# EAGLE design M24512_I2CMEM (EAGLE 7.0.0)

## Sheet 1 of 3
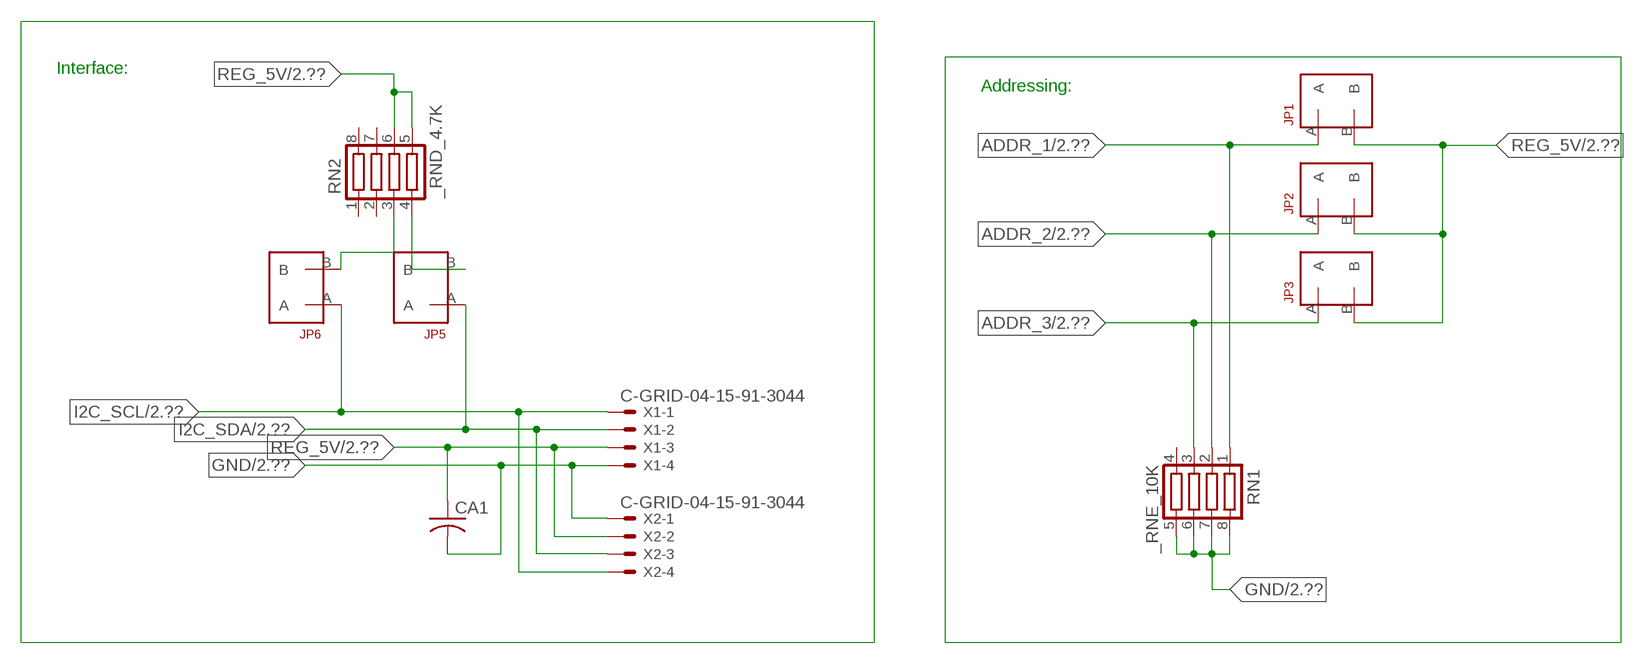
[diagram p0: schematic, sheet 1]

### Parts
CA1  CC1206KRX7R9BB104  [.1UF]
JP1  JUMPER_1X2_2MM  [JUMPER_1X2_2MM]
JP2  JUMPER_1X2_2MM  [JUMPER_1X2_2MM]
JP3  JUMPER_1X2_2MM  [JUMPER_1X2_2MM]
JP5  JUMPER_1X2_2MM  [JUMPER_1X2_2MM]
JP6  JUMPER_1X2_2MM  [JUMPER_1X2_2MM]
RN1  _RNE_10K  [RNE]
RN2  _RND_4.7K  [RND]
X1  C-GRID-04-15-91-3044  [15-91-04]
X2  C-GRID-04-15-91-3044  [15-91-04]

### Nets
ADDR_1: JP1.A RN1.1 ; also sheet 2
ADDR_2: JP2.A RN1.2 ; also sheet 2
ADDR_3: JP3.A RN1.3 ; also sheet 2
GND: CA1.2 RN1.5 RN1.6 RN1.7 RN1.8 X1.4 X2.1 ; also sheet 2,3
I2C_SCL: JP6.A X1.1 X2.4 ; also sheet 2
I2C_SDA: JP5.A X1.2 X2.3 ; also sheet 2
N$1: JP6.B RN2.3
N$2: JP5.B RN2.4
REG_5V: CA1.1 JP1.B JP2.B JP3.B RN2.5 RN2.6 X1.3 X2.2 ; also sheet 2,3
Unconnected: RN1.4 RN2.1 RN2.2 RN2.7 RN2.8

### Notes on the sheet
- Interface:
- Addressing:

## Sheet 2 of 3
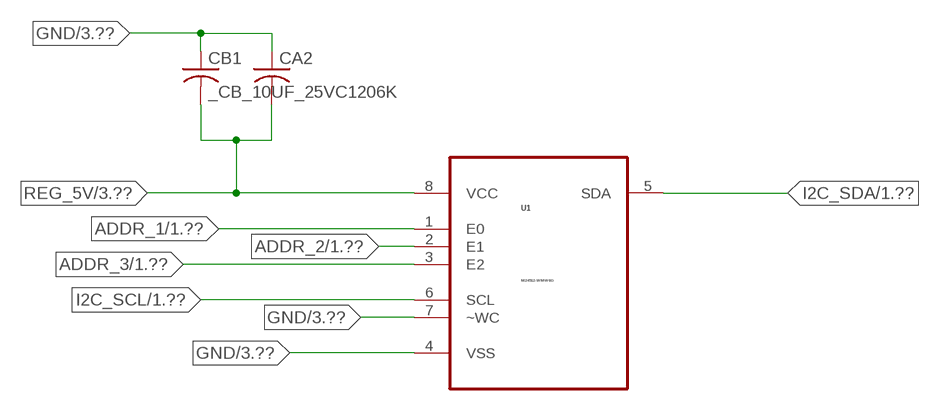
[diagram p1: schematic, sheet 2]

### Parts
CA2  _CA_.10UF_50VC1206K  [_CA_.1UF_50V]
CB1  _CB_10UF_25VC1206K  [_CB_10UF_25V]
U1  M24512-WMW6G  [SOIC127P825X250-8N]

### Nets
ADDR_1: U1.1(E0) ; also sheet 1
ADDR_2: U1.2(E1) ; also sheet 1
ADDR_3: U1.3(E2) ; also sheet 1
GND: CA2.1 CB1.1 U1.4(VSS) U1.7(~WC) ; also sheet 1,3
I2C_SCL: U1.6(SCL) ; also sheet 1
I2C_SDA: U1.5(SDA) ; also sheet 1
REG_5V: CA2.2 CB1.2 U1.8(VCC) ; also sheet 1,3

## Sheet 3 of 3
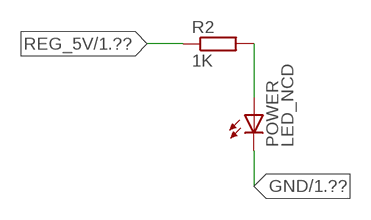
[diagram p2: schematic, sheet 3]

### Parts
POWER  LED_NCD  [CHIPLED_0603]
R2  1K  RESISTOR_SMT-0402  [R402]

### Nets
GND: POWER.C ; also sheet 1,2
N$13: POWER.A R2.2
REG_5V: R2.1 ; also sheet 1,2

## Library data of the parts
CA1 = NCD_ULTIMATE_LIBRARY:CC1206KRX7R9BB104: Capacitor CA .1uF 50V SMT C1206K CC1206KRX7R9BB104
CA2 = NCD_ULTIMATE_LIBRARY:_CA_.10UF_50V: Capacitor .1uF SMT
CB1 = NCD_ULTIMATE_LIBRARY:_CB_10UF_25V: Capacitor 10uF SMT
JP1-JP3 JP5 JP6 = NCD_ULTIMATE_CONNECTORS:JUMPER_1X2_2MM
POWER = NCD_ULTIMATE_LIBRARY:LED_NCD: LED Digikey 754-1132-2-ND/APT2012SRCPRV
R2 = NCD_ULTIMATE_LIBRARY:RESISTOR_SMT: NCD Resistor
RN1 = NCD_ULTIMATE_LIBRARY:_RNE_10K: Resistor Array RNE SMT 10K x 4 Single Resistor Source: http://www.ctscorp.com/components/Datasheets/CTSChipArrayDs.pdf Digikey 742C083103JPTR-ND/742C083103JP; OC_FARNELL: unknown; OC_NEWARK: unknown
RN2 = NCD_ULTIMATE_LIBRARY:_RND_4.7K: Resistor Array RND SMT 4.7K x 4 Single Resistor Source: http://www.ctscorp.com/components/Datasheets/CTSChipArrayDs.pdf Digikey 742C083472JPTR-ND/742C083472JP; OC_FARNELL: unknown; OC_NEWARK: unknown
U1 = NCD_ULTIMATE_bhaskar:M24512-WMW6G: Digikey 497-8625-6-ND/M24512-WDW6TP; MPN: M24512-WMW6G; OC_FARNELL: 1099661; OC_NEWARK: 56P9161; PACKAGE: SOIC-8; SUPPLIER: STMICROELECTRONICS
X1 X2 = NCD_ULTIMATE_CONNECTORS:C-GRID-04: CONNECTOR 4-Pos I2C wire to board 2.54 mm (0.100") pitch header Digikey WM1342-ND/0015912045; OC_FARNELL: unknown; OC_NEWARK: unknown

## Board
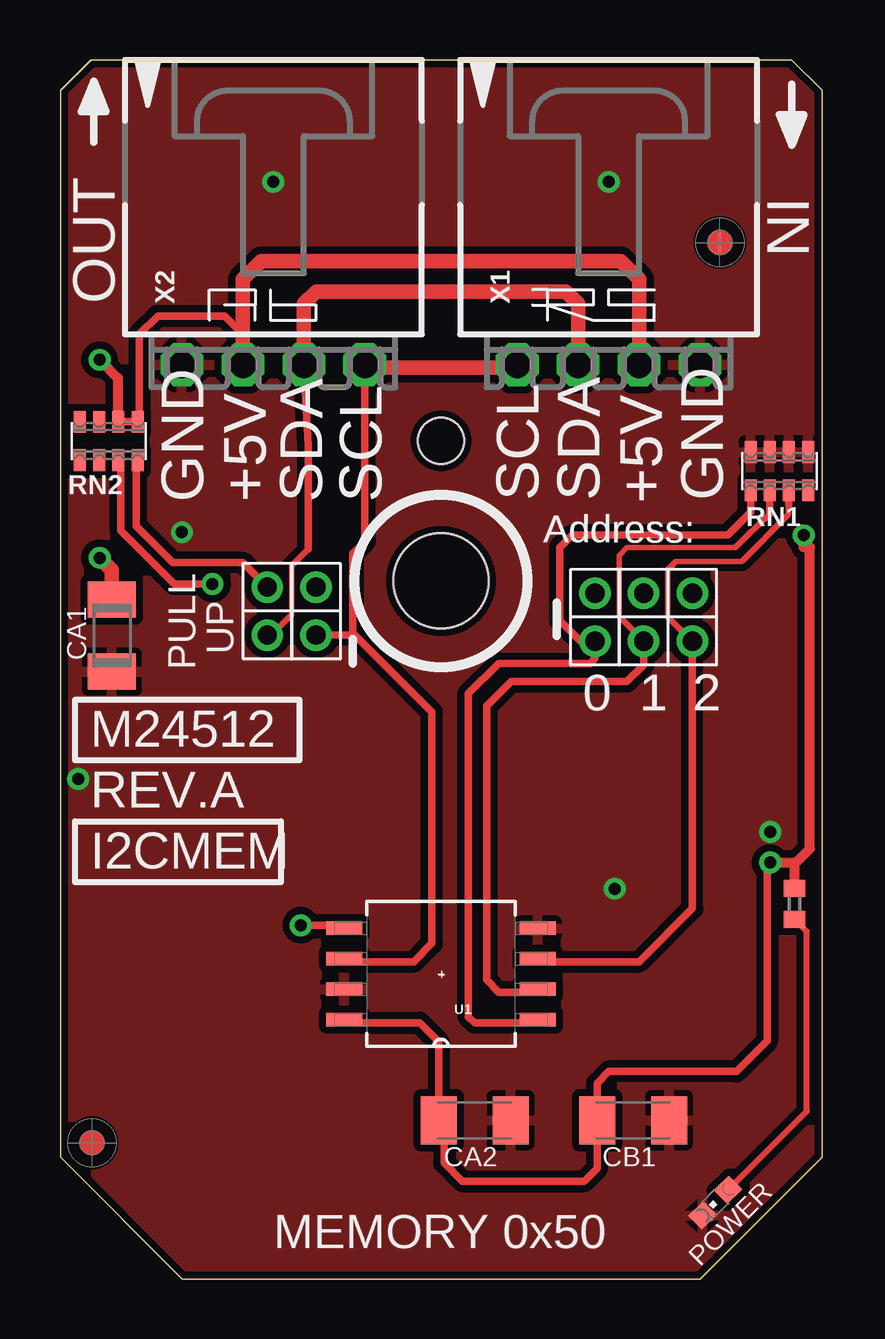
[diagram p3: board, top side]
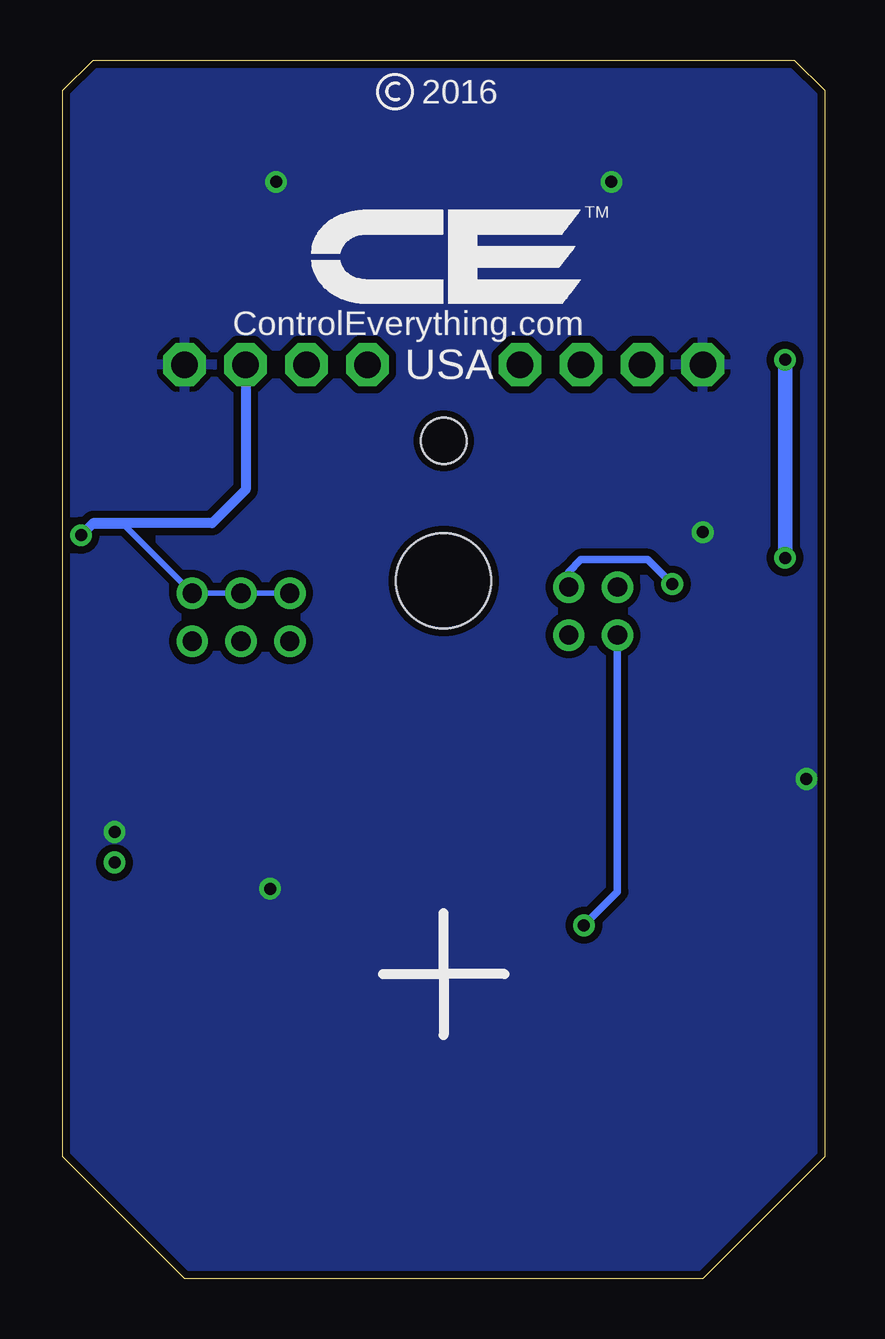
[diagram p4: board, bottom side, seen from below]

Size 31.75 x 50.8 mm. Coordinates in mm from the lower left corner, seen from the top.
Outline: 32 segments
Copper layers (1*16): Top 0.035mm / dielectric 1.5mm / Bottom 0.035mm
Design rules "default": minimum track width 5mil, minimum drill 24mil, track to track 5mil, track to pad 5mil, pad to pad 5mil, via to via 5mil, smd to smd 5mil, copper to edge 10mil, drill to drill 8mil, minimum pad ring 10mil, minimum via ring 8mil, stop-mask expansion 2mil, vias tented up to drill 0mil, thermal gap 10mil
Holes 3.96 mm at 15.88,29.08
Holes 1.91 mm at 15.88,34.92

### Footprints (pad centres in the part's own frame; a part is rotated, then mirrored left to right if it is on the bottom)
.1UF = smd 1.5 x 2: 1 -1.5,0; 2 1.5,0
_CA_.1UF_50V = smd 1.5 x 2: 1 -1.5,0; 2 1.5,0
_CB_10UF_25V = smd 1.5 x 2: 1 -1.5,0; 2 1.5,0
JUMPER_1X2_2MM = drill 0.8: A 0,2; B 0,0
CHIPLED_0603 = smd 0.8 x 0.876: A 0,-0.75; C 0,0.75
R402 = smd 0.7 x 0.9: 1 -0.65,0; 2 0.65,0
RNE = smd 0.5 x 0.9: 1 -1.2,-0.8; 2 -0.4,-0.8; 3 0.4,-0.8; 4 1.2,-0.8; 5 1.2,0.8; 6 0.4,0.8; 7 -0.4,0.8; 8 -1.2,0.8
RND = smd 0.5 x 0.9: 1 -1.2,-0.8; 2 -0.4,-0.8; 3 0.4,-0.8; 4 1.2,-0.8; 5 1.2,0.8; 6 0.4,0.8; 7 -0.4,0.8; 8 -1.2,0.8
SOIC127P825X250-8N = smd 1.499 x 0.559: 1 -4.039,1.905; 2 -4.039,0.635; 3 -4.039,-0.635; 4 -4.039,-1.905; 5 4.039,-1.905; 6 4.039,-0.635; 7 4.039,0.635; 8 4.039,1.905
15-91-04 = drill 1.1 pad 1.778 octagon: 1 -3.81,-7.62; 2 -1.27,-7.62; 3 1.27,-7.62; 4 3.81,-7.62

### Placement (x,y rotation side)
CA1  2.16,26.81 270 top
CA2  17.27,6.6 180 top
CB1  23.88,6.6 180 top
JP1  22.29,28.57 180 top
JP2  24.32,28.57 180 top
JP3  26.35,28.57 180 top
JP5  8.64,28.83 180 top
JP6  10.67,28.83 180 top
POWER  27.3,3.18 135 top
R2  30.61,15.62 270 top
RN1  29.97,33.66 0 top
RN2  2.03,34.92 0 top
U1  15.88,12.7 180 top
U$5  [VISION_REF10]  1.33,5.66 90 top
U$28  [VISION_REF10]  27.5,43.19 90 top
X1  22.86,45.72 0 top
X2  8.89,45.72 0 top

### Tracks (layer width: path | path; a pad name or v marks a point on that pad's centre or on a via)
ADDR_1
  Top 0.305: RN1.1 28.77,31.95 27.81,30.99 21.34,30.99 20.83,30.48 20.83,27.43 21.68,26.58 JP1.A 22.29,25.85 22.1,25.65 18.29,25.65 17.02,24.38 17.02,10.92 17.27,10.67 19.15,10.67 U1.1
ADDR_2
  Top 0.229: 29.57,31.9 28.14,30.48 23.62,30.48 23.29,30.15 23.29,27.61 JP2.A
  Top 0.305: RN1.2 29.57,32.11 29.57,31.9 | U1.2 19.15,11.94 18.29,11.94 17.78,12.45 17.78,23.88 18.8,24.89 23.62,24.89 24.32,25.59 JP2.A
ADDR_3
  Top 0.229: 30.37,32.28 30.35,32.26 30.35,31.85 28.4,29.9 25.65,29.9 25.32,29.57 25.32,27.58 26.33,26.58 JP3.A
  Top 0.305: RN1.3 30.37,32.28 | U1.3 20.68,13.21 24.13,13.21 26.35,15.43 JP3.A
GND  (via drill 0.5)
  other vias: 8.89,45.72 22.86,45.72 29.59,18.62 0.76,20.83 23.11,16.26 5.08,31.12
  pour Bottom (isolate 0.305): 4.45,-0.63 -0.64,4.45 -0.64,50.17 0.64,51.44 31.11,51.44 32.38,50.17 32.38,4.45 27.3,-0.63
  pour Top (isolate 0.305): 3.81,-1.27 -1.27,3.81 -1.27,50.8 0,52.07 31.75,52.07 33.02,50.8 33.02,3.81 27.94,-1.27
I2C_SCL
  Top 0.305: 12.7,37.97 12.7,30.73 12.19,30.23 12.19,26.83 | U1.6 11.96,13.21 14.73,13.21 15.49,13.97 15.49,23.62 12.29,26.83 12.19,26.83 | 12.19,26.83 JP6.A
  Top 0.406: X2.4 12.7,37.97 | 19.05,37.97 X1.1
  Top 0.61: 12.7,37.97 19.05,37.97
I2C_SDA  (via drill 0.5)
  Top 0.229: 10.35,30.42 9.65,29.72 9.65,27.69 8.79,26.83 JP5.A
  Top 0.305: 10.35,30.42 10.35,34.73 X2.3 | U1.5 11.71,14.73 v10.03,14.73
  Top 0.61: X2.3 10.16,40.64 10.67,41.15 21.08,41.15 21.59,40.64 X1.2
  Bottom 0.305: v10.03,14.73 8.64,16.13 JP5.A
N$1  (via drill 0.5)
  Top 0.305: RN2.3 2.54,34.02 2.54,31.18 4.76,28.96 v6.35,28.96
  Bottom 0.305: v6.35,28.96 7.37,29.97 10.16,29.97 10.67,29.46 JP6.B
N$2
  Top 0.305: RN2.4 3.17,34.07 3.17,31.37 4.7,29.85 7.62,29.85 JP5.B
N$13
  Top 0.254: POWER.A 31.11,6.99 31.11,14.46 R2.2
REG_5V  (via drill 0.5)
  Top 0.305: 7.62,39.37 7.49,39.37 | RN2.6 RN2.5 3.3,35.8 3.3,39.37 4.06,40.13 6.86,40.13 7.62,39.37 | X2.2 7.62,39.37 | v29.59,17.35 29.46,17.22 29.46,9.91 28.19,8.64 22.86,8.64 22.38,8.15 CB1.2 22.38,4.6 21.84,4.06 16.76,4.06 16,4.83 16,6.37 CA2.2 15.77,9.88 14.99,10.67 12.6,10.67 U1.8
  Top 0.406: v29.59,17.35 30.48,17.35 | 30.48,17.35 30.67,17.35 31.24,17.92 31.24,30.48 30.99,30.48 v30.99,30.99 | v1.65,38.3 2.41,37.54 2.41,35.74 RN2.6 | R2.1 30.61,17.22 30.48,17.35
  Top 0.61: X2.2 7.62,41.66 8.38,42.42 23.37,42.42 24.13,41.66 X1.3 | CA1.1 2.16,29.54 v1.65,30.05
  Top 0.813: v30.99,30.99 31.05,30.99
  Bottom 0.229: JP1.B JP2.B JP3.B 29.15,31.37 30.61,31.37
  Bottom 0.406: 24.13,38.23 X1.3 | X1.3 24.13,32.89 25.53,31.5 30.48,31.5 30.61,31.37 v30.99,30.99 | X1.3
  Bottom 0.61: v1.65,30.05 v1.65,38.3

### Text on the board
tNames: IN | OUT | GND | GND | +5V | +5V | SDA | SDA | SCL | SCL | SCL | SCL | SDA | SDA | +5V | +5V | GND | GND | Address: | Address: | UP | PULL | 0 | 1 | 2 | M24512 | REV.A | I2CMEM | MEMORY 0x50
bNames: 2016 | TM | ControlEverything.com | USA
